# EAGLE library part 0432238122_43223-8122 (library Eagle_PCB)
PCB terminal block - MPT 0,5/ 2-2,54 - 1725656 Check prices
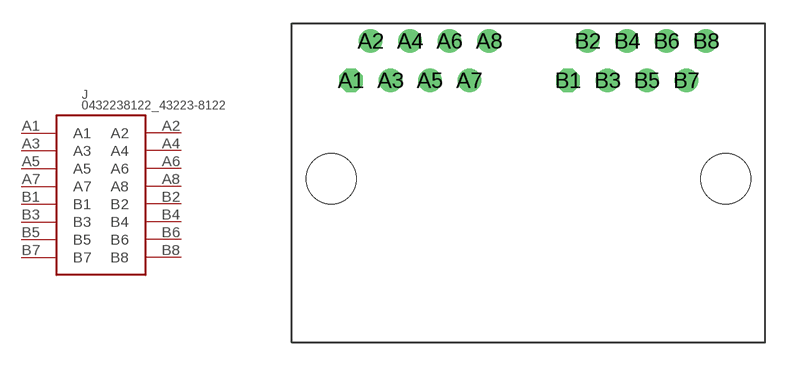
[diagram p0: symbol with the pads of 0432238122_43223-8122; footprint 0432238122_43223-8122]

Designator prefix J

## 0432238122_43223-8122 (AVAILABILITY: In Stock; DESCRIPTION: CONN MOD JACK 8P8C R/A UNSHLD; MF: Molex; MP: 0432238122; PACKAGE: None; PRICE: None)  [0432238122_43223-8122]
A1  A1
A2  A2
A3  A3
A4  A4
A5  A5
A6  A6
A7  A7
A8  A8
B1  B1
B2  B2
B3  B3
B4  B4
B5  B5
B6  B6
B7  B7
B8  B8

## Footprint 0432238122_43223-8122 (pad centres in mm)
PCB terminal block - MPT 0,5/ 3-2,54
drill 1 octagon: A1 1.27,6.35; B1 15.24,6.35
drill 1: A2 2.54,8.89; A3 3.81,6.35; A4 5.08,8.89; A5 6.35,6.35; A6 7.62,8.89; A7 8.89,6.35; A8 10.16,8.89; B2 16.51,8.89; B3 17.78,6.35; B4 19.05,8.89; B5 20.32,6.35; B6 21.59,8.89; B7 22.86,6.35; B8 24.13,8.89
hole 3.25 at 0,0
hole 3.25 at 25.4,0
